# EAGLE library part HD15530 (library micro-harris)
MICROCONTROLLER/MEMORY DEVICE
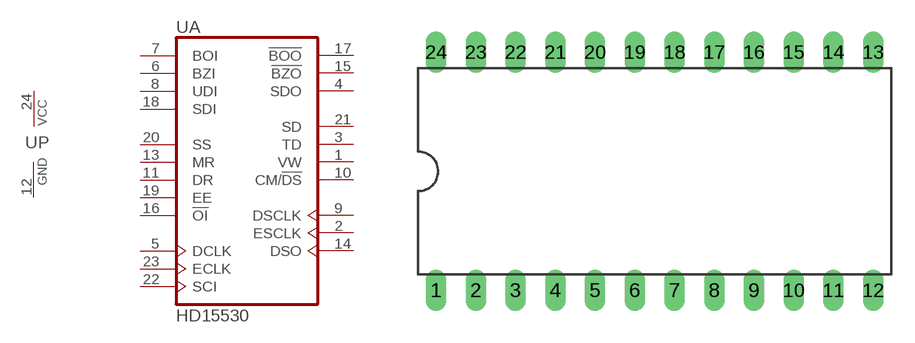
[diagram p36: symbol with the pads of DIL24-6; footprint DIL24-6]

Designator prefix U; gates A=HD15530 P=PWRN

## HD15530 (OC_FARNELL: unknown; OC_NEWARK: unknown)  [DIL24-6]
1  A:VW  out
2  A:ESCLK  out
3  A:TD  out
4  A:SDO  out
5  A:DCLK  in
6  A:BZI  in
7  A:BOI  in
8  A:UDI  in
9  A:DSCLK  out
10  A:CM/!DS  out
11  A:DR  in
12  P:GND  pwr
13  A:MR  in
14  A:DSO  out
15  A:!BZO  out
16  A:!OI  in
17  A:!BOO  out
18  A:SDI  in
19  A:EE  in
20  A:SS  in
21  A:SD  out
22  A:SCI  in
23  A:ECLK  in
24  P:VCC  pwr

## Footprint DIL24-6 (pad centres in mm)
Dual In Line Package 0.6 inch
drill 0.813 long: 1 -13.97,-7.62; 2 -11.43,-7.62; 3 -8.89,-7.62; 4 -6.35,-7.62; 5 -3.81,-7.62; 6 -1.27,-7.62; 7 1.27,-7.62; 8 3.81,-7.62; 9 6.35,-7.62; 10 8.89,-7.62; 11 11.43,-7.62; 12 13.97,-7.62; 13 13.97,7.62; 14 11.43,7.62; 15 8.89,7.62; 16 6.35,7.62; 17 3.81,7.62; 18 1.27,7.62; 19 -1.27,7.62; 20 -3.81,7.62; 21 -6.35,7.62; 22 -8.89,7.62; 23 -11.43,7.62; 24 -13.97,7.62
